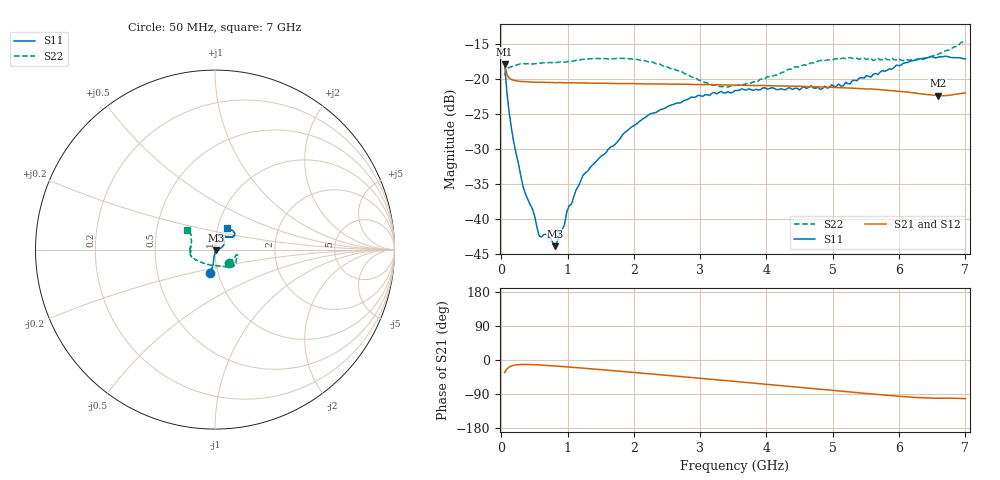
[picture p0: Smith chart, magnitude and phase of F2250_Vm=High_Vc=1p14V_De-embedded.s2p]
! Integrated Device Technology
! Corporate Headquarters
! 6024 Silver Creek Valley Road
! San Jose, CA 95138  USA
! Phone:  1-408-284-8200
! Toll Free:  1-800-223-1366
! Webpage:  http://www.idt.com/
! Timing and RF Division
! 515 Groton Road, Suite 102
! Westford, MA 01886-6024
! Device:  F2250
! Description: Voltage Variable RF Attenuator
! Frequency:  50.0 -  6000.00 MHz
! Package:  3x3 mm Thin QFN Plastic Package: 16 pin
! Ports:  2 RF, 3 DC
!  Pin  1  = GND
!  Pin  2  = NC
!  Pin  3  = RF1  = Port 1
!  Pin  4  = NC
!  Pin  5  = GND
!  Pin  6  = GND
!  Pin  7  = GND
!  Pin  8  = GND
!  Pin  9  = NC
!  Pin 10  = RF2  = Port 2
!  Pin 11  = NC
!  Pin 12  = GND
!  Pin 13  = GND
!  Pin 14  = VCNTRL
!  Pin 15  = VDD
!  Pin 16  = VMODE
! Vcntrl:  1.140 Volts
! Vmode:  +3.300 Volts
! Vdd:  +3.30  Volts
! Current:  1.330 mA
! Data:  The device was measured on a the F2250 evaluation board which has
!  individual transmission lines to the RF pins.  Data was collected
!  using a calibrated network analyzer.  The evaluation board was
!  de-embedded using a TRL calibration technique.
!  The reference plane is the edge of the package pin.
! Misc:  SN 10
!  Action Tracker AT0258
! Date Measured:  2014-11-26
! Date:  2015-10-15  MJV
! Note:
!  Integrated Device Technology supplies this data as a sample of measured
!  data at the package pin for this product.  Your particular data for this
!  product may vary.
!  Data was taken at 25 degrees C.
!  Integrated Device Technology reserves the right to change this data at anytime.
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# GHz S dB R 50
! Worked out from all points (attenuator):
!   201 points, 50 MHz to 7 GHz, reference 50 ohm
!   highest |S21| = -17.93 dB at 50 MHz (marker M1); lowest = -22.4 dB at 6.583 GHz (marker M2)
!   lowest |S11| = -43.9 dB at 814.5 MHz (marker M3), VSWR 1.01, Z = 50.6 - j0.259 ohm
!   |S11| at or under -10 dB: start of sweep to end of sweep
!   |S22| runs from -21.2 to -14.5 dB; largest |S21 - S12| = 0.00035
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0.05  -17.59 -101.5  -17.93 -33.2  -17.92 -33.2  -19.49 -44.7
0.08475  -21.95 -96.7  -19.38 -23.5  -19.37 -23.5  -18.52 -22.5
0.15425  -27.12 -98.2  -20.10 -15.6  -20.09 -15.6  -18.28 -13.8
0.328  -35.37 -89.5  -20.38 -11.8  -20.39 -11.8  -17.81 -12.8
0.467  -38.51 -86.0  -20.45 -12.2  -20.46 -12.2  -17.88 -14.9
0.57125  -42.42 -63.4  -20.49 -13.1  -20.47 -13.1  -17.79 -17.5
0.6755  -42.20 -55.2  -20.50 -14.2  -20.50 -14.2  -17.70 -19.6
0.8145  -43.89 -23.6  -20.55 -15.8  -20.54 -15.8  -17.69 -23.3
0.884  -41.73 -19.3  -20.53 -16.7  -20.55 -16.7  -17.60 -25.5
0.9535  -40.85 -25.4  -20.57 -17.6  -20.57 -17.6  -17.64 -26.8
0.98825  -38.97 -21.0  -20.56 -18.1  -20.55 -18.1  -17.57 -27.5
1.023  -38.13 -15.6  -20.55 -18.5  -20.55 -18.5  -17.49 -27.8
1.2315  -33.78 -0.5  -20.59 -21.4  -20.60 -21.5  -17.20 -32.3
1.857  -27.69 19.3  -20.67 -30.7  -20.66 -30.7  -17.08 -41.7
2.37825  -24.52 32.4  -20.72 -38.6  -20.73 -38.6  -17.82 -50.3
3.1775  -22.05 54.5  -20.83 -51.1  -20.83 -51.1  -20.86 -81.5
3.525  -21.65 64.8  -20.89 -56.5  -20.89 -56.6  -20.97 -105.7
4.7065  -21.31 68.6  -21.13 -75.4  -21.12 -75.4  -17.72 -157.5
5.15825  -21.00 52.1  -21.27 -82.7  -21.27 -82.7  -17.04 -166.4
5.85325  -18.55 37.0  -21.66 -93.6  -21.66 -93.8  -17.28 178.5
6.583  -16.92 42.6  -22.41 -100.8  -22.40 -101.0  -16.48 152.2
7  -17.15 61.9  -21.99 -101.9  -21.99 -102.1  -14.51 144.6
